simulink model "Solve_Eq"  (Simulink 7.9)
settings: Solver=ode45  StartTime=0.0  StopTime=T  RelTol=1e-3
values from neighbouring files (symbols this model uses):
  c = CModal(i,i)    [Example_4_MDOF_Random.m]    (also in Sdof_Random.m = 10)
  dt = 1/Fs    [Example_4_MDOF_Random.m]    (also in Sdof_Random.m)
  k = KModal(i,i)    [Example_4_MDOF_Random.m]    (also in Sdof_Random.m = 10000)
  m = MModal(i,i)    [Example_4_MDOF_Random.m]    (also in Sdof_Random.m = 1)

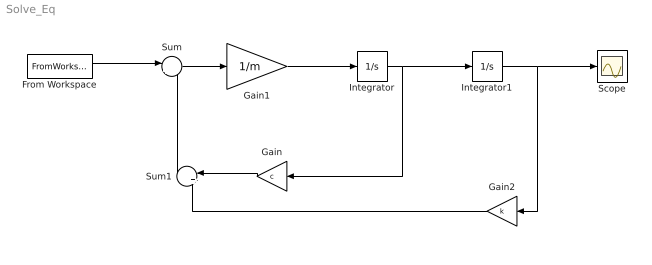
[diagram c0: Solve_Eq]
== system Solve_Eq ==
  From Workspace : FromWorkspace  VariableName=force  SampleTime=dt
  Gain : Gain  Gain=c
  Gain1 : Gain  Gain=1/m
  Gain2 : Gain  Gain=k
  Integrator : Integrator
  Integrator1 : Integrator
  Scope : Scope
  Sum : Sum  Inputs=|+-
  Sum1 : Sum  Inputs=|++
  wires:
  From Workspace/1 -> Sum/1
  Sum1/1 -> Sum/2
  Sum/1 -> Gain1/1
  Gain1/1 -> Integrator/1
  Integrator/1 -> Integrator1/1, Gain/1
  Integrator1/1 -> Scope/1, Gain2/1
  Gain/1 -> Sum1/1
  Gain2/1 -> Sum1/2
